// provides methods to be called from this PLC context as well as other PLC contexts.
// Instances have to be declared in this PLC context.
// ObjectID has to be transmitted via process image
{attribute 'c++_compatible'}
FUNCTION_BLOCK FB_Calculation EXTENDS TcBaseModuleRegistered IMPLEMENTS I_Calculation

VAR
END_VAR

{attribute 'object_name' := 'Addition'}
{attribute 'c++_compatible'}
{attribute 'signature_flag' := '33554688'}
{attribute 'pack_mode' := '4'}
{attribute 'show'}
{attribute 'minimal_input_size' := '4'}
{attribute 'checksuperglobal'}
METHOD Addition : HRESULT
VAR_INPUT
	nIn1	: INT;
	nIn2	: INT;
	nRes	: REFERENCE TO INT;
END_VAR
nRes := nIn1 + nIn2;
END_METHOD

METHOD FB_reinit : BOOL
VAR_INPUT
END_VAR
SUPER^.FB_reinit();
END_METHOD

{attribute 'object_name' := 'Subtraction'}
{attribute 'c++_compatible'}
{attribute 'signature_flag' := '33554688'}
{attribute 'pack_mode' := '4'}
{attribute 'show'}
{attribute 'minimal_input_size' := '4'}
{attribute 'checksuperglobal'}
METHOD Subtraction : HRESULT
VAR_INPUT
	nIn1	: INT;
	nIn2	: INT;
	nRes	: REFERENCE TO INT;
END_VAR
nRes := nIn1 - nIn2;
END_METHOD

{attribute 'object_name' := 'TcQueryInterface'}
{attribute 'c++_compatible'}
{attribute 'signature_flag' := '33554688'}
{attribute 'pack_mode' := '4'}
{attribute 'show'}
{attribute 'minimal_input_size' := '4'}
{attribute 'checksuperglobal'}
METHOD TcQueryInterface : HRESULT
VAR_INPUT
	iid	: REFERENCE TO IID;
	pipItf	: POINTER TO PVOID;
END_VAR

VAR
	ipCalc : I_Calculation;
	ipUnk : ITcUnknown;
END_VAR
IF GuidsEqual(ADR(iid), ADR(TC_GLOBAL_IID_LIST.IID_I_Calculation)) THEN
	ipCalc := THIS^; // cast to interface pointer
	pipItf^ := ITCUNKNOWN_TO_PVOID(ipCalc);
	TcAddRef();
	TcQueryInterface := S_OK;
ELSIF GuidsEqual(ADR(iid), ADR(TC_GLOBAL_IID_LIST.IID_ITcUnknown)) THEN
	ipUnk := THIS^; // cast to interface pointer
	pipItf^ := ITCUNKNOWN_TO_PVOID(ipUnk);
	TcAddRef(); 
	TcQueryInterface := S_OK;
ELSE
	TcQueryInterface := SUPER^.TcQueryInterface(iid, pipItf);
END_IF
END_METHOD

END_FUNCTION_BLOCK
